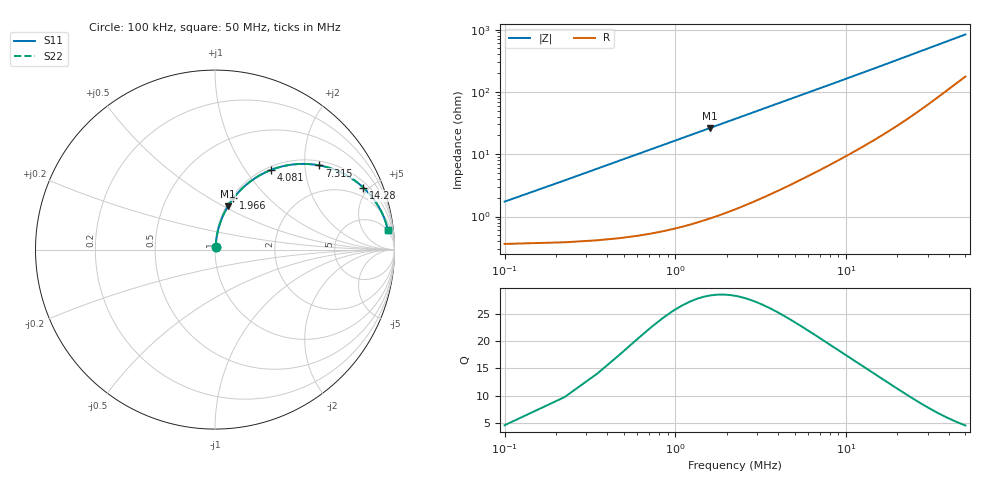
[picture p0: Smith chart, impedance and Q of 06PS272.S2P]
! Coilcraft 0603PS-272 Power Chip Inductor
! 19 February 2003
# MHZ S MA R 50
!Freq  MagS11  AngS11  MagS21  AngS21  MagS12  AngS12  MagS22  AngS22
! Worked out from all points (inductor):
!   403 points, 100 kHz to 50 MHz, reference 50 ohm
!   read as one part in series: L = 2.66 uH near 348.8 kHz
!   highest Q = 28.3 at 1.593 MHz (marker M1), where L = 2.62 uH
!   S11 on the Smith chart (normalised r, x): 100 kHz: 1.01, +0.03; 1.966 MHz: 1.02, +0.65; 4.081 MHz: 1.05, +1.33; 7.315 MHz: 1.12, +2.38; 14.28 MHz: 1.33, +4.64; 50 MHz: 5, +16
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0.1  0.01729 76.9  0.9962 -1.0  0.9962 -1.0  0.01729 76.9
0.2244  0.03778 82.0  0.9955 -2.2  0.9955 -2.2  0.03778 82.0
0.4732  0.07854 82.2  0.9925 -4.5  0.9925 -4.5  0.07854 82.2
0.5976  0.09869 81.5  0.9903 -5.7  0.9903 -5.7  0.09869 81.5
0.722  0.1187 80.6  0.9877 -6.8  0.9877 -6.8  0.1187 80.6
0.8464  0.1384 79.7  0.9847 -7.9  0.9847 -7.9  0.1384 79.7
1.0952  0.1773 77.6  0.9775 -10.2  0.9775 -10.2  0.1773 77.6
1.344  0.2152 75.5  0.9688 -12.4  0.9688 -12.4  0.2152 75.5
1.5928  0.2519 73.4  0.9589 -14.6  0.9589 -14.6  0.2519 73.4
1.966  0.3047 70.3  0.9418 -17.7  0.9418 -17.7  0.3047 70.3
2.8368  0.4159 63.3  0.8943 -24.6  0.8943 -24.6  0.4159 63.3
4.0808  0.5448 54.7  0.8171 -33.0  0.8171 -33.0  0.5448 54.7
5.4492  0.65 47.0  0.7319 -40.5  0.7319 -40.5  0.65 47.0
7.3152  0.7476 38.9  0.6282 -48.3  0.6282 -48.3  0.7476 38.9
8.4348  0.7884 35.0  0.5749 -51.9  0.5749 -51.9  0.7884 35.0
11.0472  0.8521 28.3  0.4745 -58.3  0.4745 -58.3  0.8521 28.3
14.2816  0.8961 22.6  0.3855 -63.4  0.3855 -63.4  0.8961 22.6
16.7696  0.9165 19.5  0.3352 -66.0  0.3352 -66.0  0.9165 19.5
25.1044  0.9491 13.2  0.2299 -70.7  0.2299 -70.7  0.9491 13.2
33.4392  0.9611 9.9  0.1733 -72.1  0.1733 -72.1  0.9611 9.9
41.774  0.9664 7.9  0.1387 -72.1  0.1387 -72.1  0.9664 7.9
50  0.9691 6.5  0.116 -71.3  0.116 -71.3  0.9691 6.5
